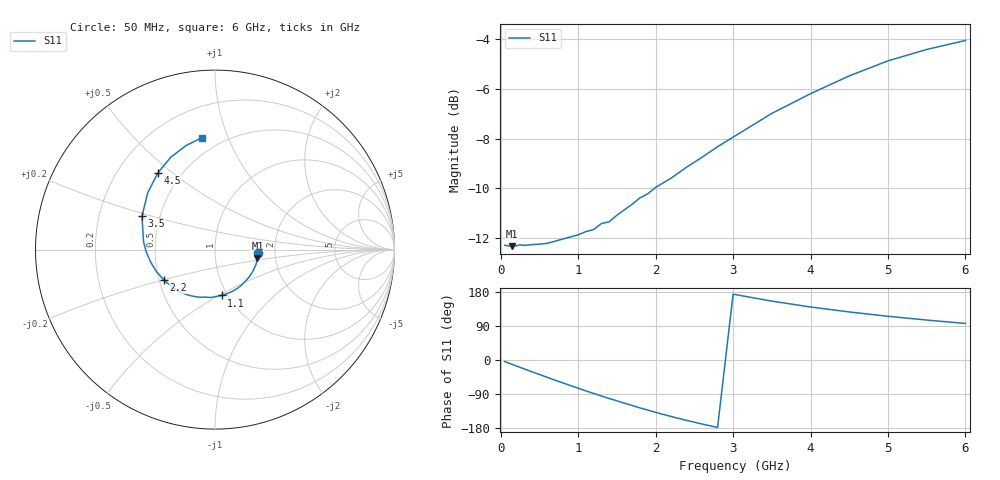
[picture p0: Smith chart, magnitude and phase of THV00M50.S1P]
! SIEMENS Discrete & RF Semiconductors
! BAS70
! Si Schottky Diode in SOT23
! IF = 0.5 mA
! S-Parameters:  February  1997
# GHz  S  MA  R  50
!  f  S11
! GHz  MAG  ANG
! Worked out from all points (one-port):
!   34 points, 50 MHz to 6 GHz, reference 50 ohm
!   lowest |S11| = -12.3 dB at 150 MHz (marker M1), VSWR 1.64, Z = 80.4 - j8.36 ohm
!   |S11| at or under -10 dB: start of sweep to 1.99 GHz
!   S11 on the Smith chart (normalised r, x): 50 MHz: 1.64, -0.06; 1.1 GHz: 0.94, -0.52; 2.2 GHz: 0.53, -0.20; 3.5 GHz: 0.40, +0.18; 4.5 GHz: 0.37, +0.44; 6 GHz: 0.39, +0.81
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0.05  0.2425 -4.1
0.15  0.2414 -11.7
0.25  0.2429 -19.4
0.4  0.243 -30.8
0.6  0.2445 -45.7
0.8  0.2495 -60.2
0.9  0.252 -67.6
1.1  0.2583 -81.6
1.2  0.2607 -88.2
1.3  0.2681 -95.0
1.4  0.2703 -101.6
1.5  0.2787 -107.7
1.6  0.286 -114.2
1.7  0.2935 -120.1
1.8  0.3023 -126.6
1.9  0.308 -132.1
2  0.3172 -138.2
2.2  0.3311 -149.1
2.4  0.3485 -159.4
2.6  0.3649 -169.0
2.8  0.3834 -178.0
3  0.4006 173.7
3.5  0.4474 155.4
4  0.4904 139.9
4.5  0.5327 126.8
5  0.5712 115.4
5.5  0.6023 105.4
6  0.6281 96.5
